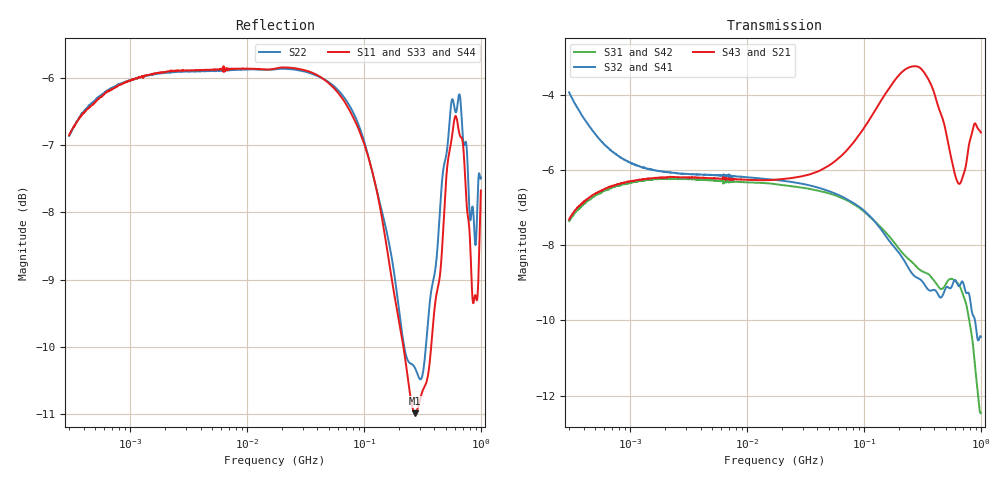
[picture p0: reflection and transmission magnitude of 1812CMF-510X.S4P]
!s-Parameter Generated by FASTRON Sdn. Bhd.
!FASTRON P/N : 1812CMF-510X
!Keysight Technologies: E5071C_MY46733604_B.14.02
!Date: Mon Mar 09 11:42:12 2026
!Version  :Rev00  Mon Mar 09 11:42:12 2026
!Data & Calibration Information:
!Freq	S11:SOLT4(ON)	S12:SOLT4(ON)	S13:SOLT4(ON)	S14:SOLT4(ON)
!	S21:SOLT4(ON)	S22:SOLT4(ON)	S23:SOLT4(ON)	S24:SOLT4(ON)
!	S31:SOLT4(ON)	S32:SOLT4(ON)	S33:SOLT4(ON)	S34:SOLT4(ON)
!	S41:SOLT4(ON)	S42:SOLT4(ON)	S43:SOLT4(ON)	S44:SOLT4(ON)
!PortZ  Port1:50+j0  Port2:50+j0  Port3:50+j0  Port4:50+j0
!When reading reference impedance value at option line is always used.
! Remarks : This data is being provided solely for informational purposes.
# Hz S dB R 50
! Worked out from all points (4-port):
!   1601 points, 300 kHz to 1 GHz, reference 50 ohm
!   strongest paths, dB at 300 kHz, 2.303 MHz, 17.55 MHz, 132.8 MHz, 1 GHz:
!     S43: -7.3, -6.2, -6.3, -4.3, -5.0
!     S21: -7.4, -6.2, -6.3, -4.3, -5.2
!     S32: -3.9, -6.1, -6.3, -7.5, -10.4
!     S41: -3.9, -6.1, -6.3, -7.5, -11.3
!     S31: -7.4, -6.2, -6.4, -7.5, -12.5
!     S42: -7.4, -6.2, -6.4, -7.5, -11.4
!   lowest |S11| = -11.0 dB at 274.5 MHz (marker M1), VSWR 1.79, Z = 86.3 - j13.3 ohm
!   |S11| at or under -10 dB: 217.3 MHz to 375.6 MHz (158.3 MHz wide, 53.4 % of centre)
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300000  -6.85 24.6  -7.39 27.5  -7.38 -152.7  -3.99 -18.8
        -7.37 27.3  -6.86 24.9  -3.93 -19.0  -7.44 -152.6
        -7.36 -152.8  -3.94 -18.9  -6.84 24.7  -7.43 27.7
        -3.90 -19.3  -7.35 -152.9  -7.32 27.2  -6.92 25.8
3324356  -5.88 2.1  -6.23 2.8  -6.22 -179.2  -6.15 -4.6
         -6.24 2.8  -5.90 2.1  -6.09 -4.6  -6.26 -179.2
         -6.25 -179.2  -6.11 -4.6  -5.88 2.0  -6.23 2.8
         -6.15 -4.5  -6.25 -179.1  -6.20 2.8  -5.89 2.0
4.268896e7  -5.99 -8.9  -6.03 5.7  -6.55 160.9  -6.52 -18.9
            -6.04 5.7  -5.99 -9.0  -6.48 -19.3  -6.60 161.4
            -6.57 160.9  -6.49 -19.4  -5.96 -9.5  -6.04 5.9
            -6.51 -18.9  -6.58 161.4  -6.01 5.8  -5.95 -8.4
2.744993e8  -10.99 -14.6  -3.31 -6.5  -8.52 79.0  -8.74 -98.7
            -3.32 -6.5  -10.32 -14.3  -8.82 -99.7  -8.68 81.9
            -8.54 79.2  -8.83 -99.7  -10.76 -18.7  -3.28 -4.9
            -8.73 -98.9  -8.67 81.7  -3.25 -4.9  -10.57 -16.2
5.597677e8  -6.93 0.8  -6.04 -19.1  -8.88 -7.3  -8.97 168.2
            -6.05 -19.0  -6.36 -4.3  -9.12 169.2  -9.21 -9.5
            -8.89 -7.2  -9.11 169.2  -7.13 -0.8  -5.73 -18.0
            -8.99 168.1  -9.21 -9.5  -5.71 -18.1  -7.08 -4.1
7.613047e8  -7.96 -7.4  -5.61 -9.7  -9.66 -77.1  -8.97 97.7
            -5.62 -9.7  -7.11 -10.0  -9.28 100.9  -9.83 -80.9
            -9.67 -77.2  -9.27 100.7  -7.29 -9.0  -5.71 -7.2
            -9.00 97.6  -9.81 -80.9  -5.69 -7.3  -7.71 -14.0
1e9  -7.67 21.9  -5.17 -24.3  -12.44 -150.8  -11.24 25.8
     -5.19 -24.1  -7.48 8.9  -10.44 30.9  -11.42 -157.3
     -12.45 -150.7  -10.44 30.8  -9.28 7.1  -5.05 -17.3
     -11.28 25.4  -11.41 -157.5  -5.01 -17.1  -7.72 10.5
